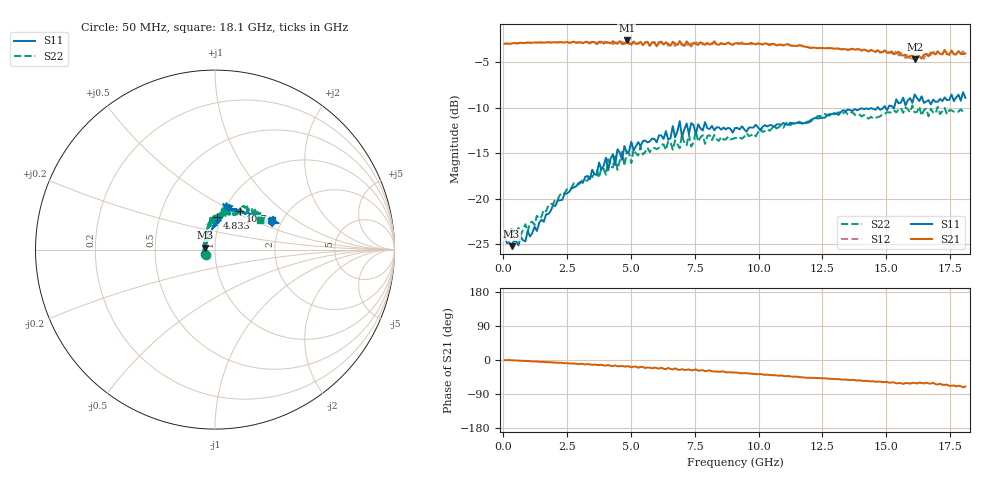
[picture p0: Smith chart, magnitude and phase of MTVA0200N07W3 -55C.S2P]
! Network Analyzer HP8720D.06.14 Serial No. US36140669
!  7 Jul 2005  07:28:53
! Frequency  S11  S21  S12  S22
# HZ  S  DB R 50
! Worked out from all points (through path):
!   201 points, 50 MHz to 18.1 GHz, reference 50 ohm
!   highest |S21| = -2.63 dB at 4.833 GHz (marker M1); lowest = -4.7 dB at 16.11 GHz (marker M2)
!   group delay of S21, straight-line fit = 10.9 ps
!   lowest |S11| = -25.2 dB at 320.8 MHz (marker M3), VSWR 1.12, Z = 44.9 + j1.05 ohm
!   |S11| at or under -10 dB: start of sweep to 14.65 GHz; 14.69 GHz to 14.89 GHz (198 MHz wide, 1.34 % of centre); 14.98 GHz to 15.08 GHz (105.3 MHz wide, 0.701 % of centre)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
!   |S22| runs from -24.2 to -9.8 dB; largest |S21 - S12| = 0.043
!   S11 on the Smith chart (normalised r, x): 50 MHz: 0.89, -0.05; 4.833 GHz: 0.96, +0.35; 10.7 GHz: 1.19, +0.54; 18.1 GHz: 1.78, +0.66
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5e7  -24.15 -155.5  -3.00 -0.5  -2.98 -0.3  -24.17 -148.7
3.2075e8  -25.19 167.8  -2.98 -0.7  -2.97 -0.9  -23.33 169.6
9.525e8  -23.54 136.7  -2.85 -2.8  -2.90 -2.6  -23.61 145.6
3.1185e9  -18.24 94.4  -2.92 -10.4  -2.93 -11.0  -17.89 109.2
4.021e9  -15.48 87.6  -2.79 -14.7  -2.92 -13.5  -17.36 100.1
4.382e9  -16.28 83.9  -2.93 -14.3  -2.85 -16.2  -15.33 98.7
4.47225e9  -14.56 79.1  -2.99 -16.4  -2.83 -14.7  -16.82 102.4
4.65275e9  -15.72 78.8  -3.03 -15.5  -2.76 -16.9  -14.84 100.2
4.743e9  -14.20 81.0  -3.00 -17.4  -2.98 -16.0  -16.40 96.4
4.83325e9  -14.92 86.4  -2.63 -16.7  -2.88 -18.2  -14.97 89.3
6.09675e9  -13.04 75.9  -2.86 -22.5  -2.77 -22.0  -14.40 85.7
6.7285e9  -13.27 80.0  -2.95 -22.2  -3.25 -23.6  -13.59 77.8
6.909e9  -11.47 76.1  -2.70 -26.2  -2.89 -24.0  -14.44 77.6
6.99925e9  -13.22 75.7  -3.05 -24.2  -3.17 -26.8  -12.94 77.3
7.17975e9  -11.73 79.8  -2.73 -26.0  -3.11 -24.7  -14.12 72.4
7.54075e9  -12.91 70.5  -3.03 -25.0  -2.82 -28.2  -12.60 79.7
9.075e9  -12.24 68.8  -2.95 -33.1  -2.92 -33.1  -13.31 66.6
1.06995e10  -11.85 57.1  -3.18 -40.9  -3.09 -40.7  -12.28 57.1
1.21435e10  -11.19 48.5  -3.41 -47.0  -3.35 -47.0  -11.22 58.5
1.512175e10  -9.78 27.0  -3.99 -60.0  -3.72 -59.5  -10.51 47.4
1.61145e10  -8.54 24.9  -4.68 -60.6  -4.18 -60.6  -10.53 41.9
1.81e10  -8.93 27.1  -4.07 -70.1  -4.40 -70.1  -10.46 32.9
